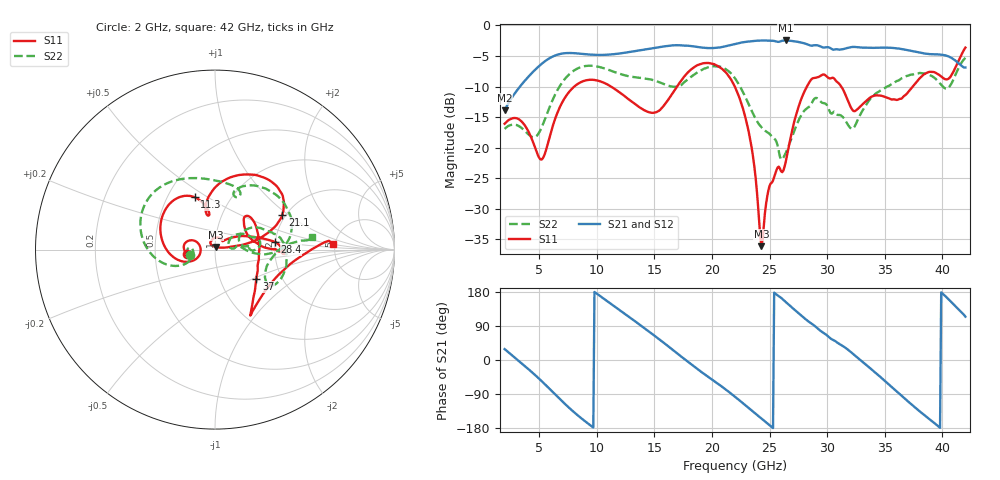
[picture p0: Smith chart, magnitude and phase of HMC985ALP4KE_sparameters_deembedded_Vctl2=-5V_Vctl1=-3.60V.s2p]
!s2p File: Measurements: S11, S21, S12, S22
# GHz S dB R 50.0
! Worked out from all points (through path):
!   401 points, 2 GHz to 42 GHz, reference 50 ohm
!   highest |S21| = -2.46 dB at 26.4 GHz (marker M1); lowest = -13.9 dB at 2 GHz (marker M2)
!   lowest |S11| = -36.1 dB at 24.3 GHz (marker M3), VSWR 1.03, Z = 50.3 + j1.54 ohm
!   |S11| at or under -10 dB: start of sweep to 8.047 GHz; 21.98 GHz to 28.25 GHz (6.264 GHz wide, 24.9 % of centre); 31.22 GHz to 37.43 GHz (6.209 GHz wide, 18.1 % of centre)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
!   |S22| runs from -21.9 to -5.3 dB; largest |S21 - S12| = 0.00061
!   S11 on the Smith chart (normalised r, x): 2 GHz: 0.73, -0.04; 11.3 GHz: 0.68, +0.44; 21.1 GHz: 1.92, +0.90; 28.4 GHz: 1.99, +0.19; 37 GHz: 1.49, -0.53; 42 GHz: 4.80, +0.50
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2  -16.09 -170.2  -13.88 28.9  -13.89 28.9  -16.93 -167.3
3.4  -15.59 165.4  -9.85 -6.9  -9.85 -6.9  -16.67 176.4
5.2  -21.96 -177.6  -6.31 -55.2  -6.31 -55.2  -16.76 -158.1
6.8  -13.34 -164.7  -4.68 -103.1  -4.68 -103.1  -9.90 -169.0
8.7  -9.21 148.3  -4.65 -154.8  -4.65 -154.8  -6.78 152.3
11.3  -10.07 111.3  -4.74 146.7  -4.74 146.7  -7.46 110.1
13.5  -13.10 99.8  -4.15 98.3  -4.15 98.3  -8.53 80.0
15.4  -13.97 103.2  -3.57 55.1  -3.57 55.1  -9.28 65.6
17.9  -7.71 77.9  -3.32 -4.5  -3.32 -4.4  -8.84 69.8
21.1  -7.50 27.3  -3.44 -75.6  -3.44 -75.6  -7.05 15.6
22  -10.07 17.8  -3.03 -97.0  -3.03 -97.0  -8.66 1.1
23.3  -18.48 9.8  -2.61 -129.3  -2.61 -129.2  -13.37 -5.0
24.3  -36.12 78.6  -2.48 -154.3  -2.48 -154.3  -16.68 5.4
25  -26.25 121.8  -2.51 -172.1  -2.51 -172.1  -17.74 8.7
26.4  -22.36 43.9  -2.46 153.2  -2.46 153.2  -20.89 30.5
28.4  -9.47 7.3  -3.18 101.2  -3.18 101.2  -13.37 18.6
28.7  -8.70 2.2  -3.31 95.1  -3.31 95.1  -12.57 17.1
32.4  -14.03 29.0  -3.52 12.0  -3.53 12.0  -16.49 26.4
35.4  -11.96 16.0  -3.65 -65.7  -3.65 -65.7  -9.85 17.8
37  -10.98 -35.3  -4.05 -108.8  -4.05 -108.7  -8.24 4.1
39.8  -8.21 -54.8  -4.77 -178.9  -4.77 -178.8  -9.50 -31.9
42  -3.63 2.6  -6.89 114.3  -6.89 114.4  -5.28 7.6
